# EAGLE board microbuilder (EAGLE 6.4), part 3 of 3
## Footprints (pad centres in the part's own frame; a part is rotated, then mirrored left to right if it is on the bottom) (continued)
TSSOP28 = smd 0.305 x 0.991: 1 -4.225,-2.918; 2 -3.575,-2.918; 3 -2.925,-2.918; 4 -2.275,-2.918; 5 -1.625,-2.918; 6 -0.975,-2.918; 7 -0.325,-2.918; 8 0.325,-2.918; 9 0.975,-2.918; 10 1.625,-2.918; 11 2.275,-2.918; 12 2.925,-2.918; 13 3.575,-2.918; 14 4.225,-2.918; 15 4.225,2.918; 16 3.575,2.918; 17 2.925,2.918; 18 2.275,2.918; 19 1.625,2.918; 20 0.975,2.918; 21 0.325,2.918; 22 -0.325,2.918; 23 -0.975,2.918; 24 -1.625,2.918; 25 -2.275,2.918; 26 -2.925,2.918; 27 -3.575,2.918; 28 -4.225,2.918
U.FL = smd 2.2 x 1.05: 1 0,1.375; 2 0,-1.375 | smd 1.05 x 1: 3 1.525,0
UG-2832HSWEG02_WRAPUNDER = smd 3.2 x 0.35 bottom: 1 -2.03,-4.03; 2 -2.03,-3.41; 3 -2.03,-2.79; 4 -2.03,-2.17; 5 -2.03,-1.55; 6 -2.03,-0.93; 7 -2.03,-0.31; 8 -2.03,0.31; 9 -2.03,0.93; 10 -2.03,1.55; 11 -2.03,2.17; 12 -2.03,2.79; 13 -2.03,3.41; 14 -2.03,4.03
UG-2832HSWEG04 = smd 2.6 x 0.35: 1 15.8,-4.55; 2 15.8,-3.9; 3 15.8,-3.25; 4 15.8,-2.6; 5 15.8,-1.95; 6 15.8,-1.3; 7 15.8,-0.65; 8 15.8,0; 9 15.8,0.65; 10 15.8,1.3; 11 15.8,1.95; 12 15.8,2.6; 13 15.8,3.25; 14 15.8,3.9; 15 15.8,4.55
UG-2832HSWEG04_WRAPAROUND = smd 2.6 x 0.35 bottom: 1 -7.7,-4.55; 2 -7.7,-3.9; 3 -7.7,-3.25; 4 -7.7,-2.6; 5 -7.7,-1.95; 6 -7.7,-1.3; 7 -7.7,-0.65; 8 -7.7,0; 9 -7.7,0.65; 10 -7.7,1.3; 11 -7.7,1.95; 12 -7.7,2.6; 13 -7.7,3.25; 14 -7.7,3.9; 15 -7.7,4.55 | hole 0.8: -2.4,4.625; -2.4,-4.625
UG-2864HSWEG01_0.96IN_WRAPAROUND = smd 0.35 x 2.2 bottom: 1 -10.15,-1.2; 2 -9.45,-1.2; 3 -8.75,-1.2; 4 -8.05,-1.2; 5 -7.35,-1.2; 6 -6.65,-1.2; 7 -5.95,-1.2; 8 -5.25,-1.2; 9 -4.55,-1.2; 10 -3.85,-1.2; 11 -3.15,-1.2; 12 -2.45,-1.2; 13 -1.75,-1.2; 14 -1.05,-1.2; 15 -0.35,-1.2; 16 0.35,-1.2; 17 1.05,-1.2; 18 1.75,-1.2; 19 2.45,-1.2; 20 3.15,-1.2; 21 3.85,-1.2; 22 4.55,-1.2; 23 5.25,-1.2; 24 5.95,-1.2; 25 6.65,-1.2; 26 7.35,-1.2; 27 8.05,-1.2; 28 8.75,-1.2; 29 9.45,-1.2; 30 10.15,-1.2 | hole 0.4: -8,-5.45; 8,-5.45
UG-2864HSWEG01_1.3_WRAPAROUND = smd 0.35 x 2.2 bottom: 1 -10.15,-0.2; 2 -9.45,-0.2; 3 -8.75,-0.2; 4 -8.05,-0.2; 5 -7.35,-0.2; 6 -6.65,-0.2; 7 -5.95,-0.2; 8 -5.25,-0.2; 9 -4.55,-0.2; 10 -3.85,-0.2; 11 -3.15,-0.2; 12 -2.45,-0.2; 13 -1.75,-0.2; 14 -1.05,-0.2; 15 -0.35,-0.2; 16 0.35,-0.2; 17 1.05,-0.2; 18 1.75,-0.2; 19 2.45,-0.2; 20 3.15,-0.2; 21 3.85,-0.2; 22 4.55,-0.2; 23 5.25,-0.2; 24 5.95,-0.2; 25 6.65,-0.2; 26 7.35,-0.2; 27 8.05,-0.2; 28 8.75,-0.2; 29 9.45,-0.2; 30 10.15,-0.2 | hole 0.4: -8,-4.45; 8,-4.45
UG-9616GLBBG02 = smd 3.5 x 0.254: 1 8.25,-3.25; 2 8.25,-2.75; 3 8.25,-2.25; 4 8.25,-1.75; 5 8.25,-1.25; 6 8.25,-0.75; 7 8.25,-0.25; 8 8.25,0.25; 9 8.25,0.75; 10 8.25,1.25; 11 8.25,1.75; 12 8.25,2.25; 13 8.25,2.75; 14 8.25,3.25
UG-9616GLBBG02_0.65MM_WRAPAROUND = smd 3.5 x 0.3 bottom: 1 -5.75,-4.225; 2 -5.75,-3.575; 3 -5.75,-2.925; 4 -5.75,-2.275; 5 -5.75,-1.625; 6 -5.75,-0.975; 7 -5.75,-0.325; 8 -5.75,0.325; 9 -5.75,0.975; 10 -5.75,1.625; 11 -5.75,2.275; 12 -5.75,3.575; 13 -5.75,2.925; 14 -5.75,4.225
UG-9616GLBBG02_WRAPAROUND = smd 3.5 x 0.254 bottom: 1 -3.75,-3.25; 2 -3.75,-2.75; 3 -3.75,-2.25; 4 -3.75,-1.75; 5 -3.75,-1.25; 6 -3.75,-0.75; 7 -3.75,-0.25; 8 -3.75,0.25; 9 -3.75,0.75; 10 -3.75,1.25; 11 -3.75,1.75; 12 -3.75,2.25; 13 -3.75,2.75; 14 -3.75,3.25
UG-9664HDDAG01 = smd 0.4 x 3: 1 -7.7,0.7; 2 -7,0.7; 3 -6.3,0.7; 4 -5.6,0.7; 5 -4.9,0.7; 6 -4.2,0.7; 7 -3.5,0.7; 8 -2.8,0.7; 9 -2.1,0.7; 10 -1.4,0.7; 11 -0.7,0.7; 12 0,0.7; 13 0.7,0.7; 14 1.4,0.7; 15 2.1,0.7; 16 2.8,0.7; 17 3.5,0.7; 18 4.2,0.7; 19 4.9,0.7; 20 5.6,0.7; 21 6.3,0.7; 22 7,0.7; 23 7.7,0.7
UG-9664HDDAG01_WRAPAROUND = smd 0.35 x 3 bottom: 1 -7.7,4.9; 2 -7,4.9; 3 -6.3,4.9; 4 -5.6,4.9; 5 -4.9,4.9; 6 -4.2,4.9; 7 -3.5,4.9; 8 -2.8,4.9; 9 -2.1,4.9; 10 -1.4,4.9; 11 -0.7,4.9; 12 0,4.9; 13 0.7,4.9; 14 1.4,4.9; 15 2.1,4.9; 16 2.8,4.9; 17 3.5,4.9; 18 4.2,4.9; 19 4.9,4.9; 20 5.6,4.9; 21 6.3,4.9; 22 7,4.9; 23 7.7,4.9 | hole 1: -8,1.45; 8,1.45
UG-9664HDDAG01_WRAPAROUND_NOHOLES = smd 0.35 x 3 bottom: 1 -7.7,4.9; 2 -7,4.9; 3 -6.3,4.9; 4 -5.6,4.9; 5 -4.9,4.9; 6 -4.2,4.9; 7 -3.5,4.9; 8 -2.8,4.9; 9 -2.1,4.9; 10 -1.4,4.9; 11 -0.7,4.9; 12 0,4.9; 13 0.7,4.9; 14 1.4,4.9; 15 2.1,4.9; 16 2.8,4.9; 17 3.5,4.9; 18 4.2,4.9; 19 4.9,4.9; 20 5.6,4.9; 21 6.3,4.9; 22 7,4.9; 23 7.7,4.9
UMAX10 = smd 0.29 x 0.9: 1 -1,-2.25; 2 -0.5,-2.25; 3 0,-2.25; 4 0.5,-2.25; 5 1,-2.25; 6 1,2.25; 7 0.5,2.25; 8 0,2.25; 9 -0.5,2.25; 10 -1,2.25
USB-MINIB = smd 0.5 x 2.308: D+ 0,4.064; D- -0.8,4.064; GND 1.6,4.064; ID 0.8,4.064; VBUS -1.6,4.064 | smd 2 x 2.4: GND1 -4.4,-2; GND2 -4.4,3.5; GND3 4.4,3.5; GND4 4.4,-2 | hole 1: -2.2,1; 2.2,1
USB-MINIB_LARGER = smd 0.5 x 2.308: D+ 0,4.064; D- -0.8,4.064; GND 1.6,4.064; ID 0.8,4.064; VBUS -1.6,4.064 | smd 2.54 x 3.81: GND1 -4.4,-2; GND4 4.4,-2 | smd 2 x 2.4: GND2 -4.4,3.5; GND3 4.4,3.5 | hole 1: -2.2,1; 2.2,1
USB_A-SMT = drill 2.5 pad 3.302: D1 -5.85,2.958; D2 5.85,2.958 | drill 1: D3 -2.25,3; D4 2.25,3 | smd 0.8 x 2.5: D+ 1,0; D- -1,0; GND 3.5,0; VBUS -3.5,0
USB_HOST-PTH = drill 0.95 long: D+ 1,6.52; D- -1,6.52; GND 3.5,6.52; VBUS -3.5,6.52 | drill 2.3 pad 2.9: S1 -6.57,3.81; S2 6.57,3.81
VCNL4000 = smd 0.35 x 0.805: 1 -1.5,-1.772; 2 -0.75,-1.772; 3 0,-1.772; 4 0.75,-1.772; 5 1.5,-1.772; 7 1.5,1.772; 8 0.75,1.772; 9 0,1.772; 10 -0.75,1.772; 11 -1.5,1.772 | smd 0.805 x 0.4: 6 1.772,-0.715; 12 -1.772,-0.2
VFBGA54 = smd 0.34 x 0.34: A1 -3.2,3.2; A2 -2.4,3.2; A3 -1.6,3.2; A7 1.6,3.2; A8 2.4,3.2; A9 3.2,3.2; B1 -3.2,2.4; B2 -2.4,2.4; B3 -1.6,2.4; B7 1.6,2.4; B8 2.4,2.4; B9 3.2,2.4; C1 -3.2,1.6; C2 -2.4,1.6; C3 -1.6,1.6; C7 1.6,1.6; C8 2.4,1.6; C9 3.2,1.6; D1 -3.2,0.8; D2 -2.4,0.8; D3 -1.6,0.8; D7 1.6,0.8; D8 2.4,0.8; D9 3.2,0.8; E1 -3.2,0; E2 -2.4,0; E3 -1.6,0; E7 1.6,0; E8 2.4,0; E9 3.2,0; F1 -3.2,-0.8; F2 -2.4,-0.8; F3 -1.6,-0.8; F7 1.6,-0.8; F8 2.4,-0.8; F9 3.2,-0.8; G1 -3.2,-1.6; G2 -2.4,-1.6; G3 -1.6,-1.6; G7 1.6,-1.6; G8 2.4,-1.6; G9 3.2,-1.6; H1 -3.2,-2.4; H2 -2.4,-2.4; H3 -1.6,-2.4; H7 1.6,-2.4; H8 2.4,-2.4; H9 3.2,-2.4; J1 -3.2,-3.2; J2 -2.4,-3.2; J3 -1.6,-3.2; J7 1.6,-3.2; J8 2.4,-3.2; J9 3.2,-3.2
VFSOP-8 = smd 0.25 x 0.65: 1 -0.75,-1.45; 2 -0.25,-1.45; 3 0.25,-1.45; 4 0.75,-1.45; 5 0.75,1.45; 6 0.25,1.45; 7 -0.25,1.45; 8 -0.75,1.45
WFDFN-14 = smd 0.2 x 0.6: P$1 -1.2,-1.5; P$2 -0.8,-1.5; P$3 -0.4,-1.5; P$4 0,-1.5; P$5 0.4,-1.5; P$6 0.8,-1.5; P$7 1.2,-1.5; P$8 1.2,1.5; P$9 0.8,1.5; P$10 0.4,1.5; P$11 0,1.5; P$12 -0.4,1.5; P$13 -0.8,1.5; P$14 -1.2,1.5 | smd 2.3 x 1.7: P$THERM 0,0
WLCSP16 = smd 0.35 x 0.35: A1 -0.75,0.75; A2 -0.25,0.75; A3 0.25,0.75; A4 0.75,0.75; B1 -0.75,0.25; B2 -0.25,0.25; B3 0.25,0.25; B4 0.75,0.25; C1 -0.75,-0.25; C2 -0.25,-0.25; C3 0.25,-0.25; C4 0.75,-0.25; D1 -0.75,-0.75; D2 -0.25,-0.75; D3 0.25,-0.75; D4 0.75,-0.75
WQFN16 = smd 0.28 x 0.85: P$1 -0.75,-1.475; P$2 -0.25,-1.475; P$3 0.25,-1.475; P$4 0.75,-1.475; P$9 0.75,1.475; P$10 0.25,1.475; P$11 -0.25,1.475; P$12 -0.75,1.475 | smd 0.85 x 0.28: P$5 1.475,-0.75; P$6 1.475,-0.25; P$7 1.475,0.25; P$8 1.475,0.75; P$13 -1.475,0.75; P$14 -1.475,0.25; P$15 -1.475,-0.25; P$16 -1.475,-0.75 | smd 1.65 x 1.65: P$17 0,0
WQFN20 = smd 0.28 x 0.85: 1 -1,-1.975; 2 -0.5,-1.975; 3 0,-1.975; 4 0.5,-1.975; 5 1,-1.975; 11 1,1.975; 12 0.5,1.975; 13 0,1.975; 14 -0.5,1.975; 15 -1,1.975 | smd 0.85 x 0.28: 6 1.975,-1; 7 1.975,-0.5; 8 1.975,0; 9 1.975,0.5; 10 1.975,1; 16 -1.975,1; 17 -1.975,0.5; 18 -1.975,0; 19 -1.975,-0.5; 20 -1.975,-1 | smd 2.65 x 2.65: 21 0,0
XBEE = drill 0.8 pad 1.27: 1 -11,9; 2 -11,7; 3 -11,5; 4 -11,3; 5 -11,1; 6 -11,-1; 7 -11,-3; 8 -11,-5; 9 -11,-7; 10 -11,-9; 11 11,-9; 12 11,-7; 13 11,-5; 14 11,-3; 15 11,-1; 16 11,1; 17 11,3; 18 11,5; 19 11,7; 20 11,9
XBEE-PRO = drill 0.8 pad 1.27: 1 -11,9; 2 -11,7; 3 -11,5; 4 -11,3; 5 -11,1; 6 -11,-1; 7 -11,-3; 8 -11,-5; 9 -11,-7; 10 -11,-9; 11 11,-9; 12 11,-7; 13 11,-5; 14 11,-3; 15 11,-1; 16 11,1; 17 11,3; 18 11,5; 19 11,7; 20 11,9
_0402 = smd 0.6 x 0.6: 1 -0.508,0; 2 0.508,0
_0402MP = smd 0.5 x 0.5: 1 -0.508,0; 2 0.508,0
_0603 = smd 0.9 x 0.8: 1 -0.762,0; 2 0.762,0
_0603MP = smd 0.8 x 0.8: 1 -0.762,0; 2 0.762,0
_0805 = smd 1.2 x 1.3: 1 -1.016,0; 2 1.016,0
_0805MP = smd 1.2 x 1.3: 1 -1.016,0; 2 1.016,0

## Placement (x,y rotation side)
0  [1X01_2MM]  not placed on the board
1  [1X01_2MM_OVAL]  not placed on the board
2  [1X01_OVAL]  not placed on the board
3  [1X01_ROUND]  not placed on the board
4  [1X02_OVAL]  not placed on the board
5  [1X02_ROUND]  not placed on the board
6  [1X02_SMT]  not placed on the board
7  [1X03_1.0MM]  not placed on the board
8  [1X03_OVAL]  not placed on the board
9  [1X03_ROUND]  not placed on the board
10  [1X03_ROUND_76]  not placed on the board
11  [1X03_SMT]  not placed on the board
12  [1X04_1.0MM]  not placed on the board
13  [1X04_OVAL]  not placed on the board
14  [1X04_ROUND]  not placed on the board
15  [1X04_ROUND_76]  not placed on the board
16  [1X04_SMT]  not placed on the board
17  [1X05_1.27MM]  not placed on the board
18  [1X05_OVAL]  not placed on the board
19  [1X05_ROUND]  not placed on the board
20  [1X05_ROUND_70]  not placed on the board
21  [1X05_ROUND_76]  not placed on the board
22  [1X05_SMT]  not placed on the board
23  [1X06_OVAL]  not placed on the board
24  [1X06_ROUND]  not placed on the board
25  [1X06_ROUND_70]  not placed on the board
26  [1X06_ROUND_76]  not placed on the board
27  [1X06_SMT]  not placed on the board
28  [1X07_OVAL]  not placed on the board
29  [1X07_ROUND]  not placed on the board
30  [1X07_ROUND_70]  not placed on the board
31  [1X07_ROUND_76]  not placed on the board
32  [1X08_OVAL]  not placed on the board
33  [1X08_ROUND]  not placed on the board
34  [1X08_ROUND_70]  not placed on the board
35  [1X08_ROUND_76]  not placed on the board
36  [1X09_OVAL]  not placed on the board
37  [1X09_ROUND_70]  not placed on the board
38  [1X09_ROUND_76]  not placed on the board
39  [1X10_OVAL]  not placed on the board
40  [1X10_ROUND]  not placed on the board
41  [1X10_ROUND70]  not placed on the board
42  [1X10_ROUND_2MM]  not placed on the board
43  [1X10_ROUND_76]  not placed on the board
44  [1X10_SMT]  not placed on the board
45  [1X11_ROUND]  not placed on the board
46  [1X11_ROUND_76]  not placed on the board
47  [1X12_OVAL]  not placed on the board
48  [1X12_ROUND]  not placed on the board
49  [1X12_ROUND_76MIL]  not placed on the board
50  [1X12_ROUND_80MIL]  not placed on the board
51  [1X13_ROUND_70]  not placed on the board
52  [1X15_ROUND_70]  not placed on the board
53  [1X16_2MM]  not placed on the board
54  [1X16_2MM_OVAL]  not placed on the board
55  [1X16_OVAL]  not placed on the board
56  [1X16_ROUND]  not placed on the board
57  [1X17_ROUND70]  not placed on the board
58  [1X20_ROUND]  not placed on the board
59  [1X23_ROUND_70MIL]  not placed on the board
60  [1X27_OVAL]  not placed on the board
61  [1X27_ROUND]  not placed on the board
62  [1X28_OVAL]  not placed on the board
63  [2X03_ROUND_70MIL]  not placed on the board
64  [2X05]  not placed on the board
65  [2X05_1.27MM_SMT]  not placed on the board
66  [2X07]  not placed on the board
67  [2X08]  not placed on the board
68  [2X10]  not placed on the board
69  [2X13]  not placed on the board
70  [2X15]  not placed on the board
71  [2X16]  not placed on the board
72  [2X23]  not placed on the board
73  [3X04]  not placed on the board
74  [3X08]  not placed on the board
75  [4UCONN_05550]  not placed on the board
76  [4UCONN_19269]  not placed on the board
77  [4UCONN_19621]  not placed on the board
78  [4UCONN_19621_SPARK]  not placed on the board
79  [32QN2]  not placed on the board
80  [869MHZANTENNA]  not placed on the board
81  [0402]  not placed on the board
82  [0603]  not placed on the board
83  [0603-MINI]  not placed on the board
84  [0805]  not placed on the board
85  [0805-THM]  not placed on the board
86  [0805_NOTHERMALS]  not placed on the board
87  [1206]  not placed on the board
88  [2012]  not placed on the board
89  [2512]  not placed on the board
90  [ADAFRUIT_2.5MM]  not placed on the board
91  [ADAFRUIT_3.5MM]  not placed on the board
92  [ADAFRUIT_5MM]  not placed on the board
93  [ADAFRUIT_9MM]  not placed on the board
94  [ADAFRUIT_16MM]  not placed on the board
95  [ADAFRUIT_30MM]  not placed on the board
96  [ADAFRUIT_TEXT_20MM]  not placed on the board
97  [ADAFRUIT_TEXT_30MM]  not placed on the board
98  [ADBM-A350]  not placed on the board
99  [ALTOIDSMINTS]  not placed on the board
100  [ANT_868MHZ_SPLATCH]  0,0 0 top
101  [ARDUINO]  25.4,0 0 top
102  [ARDUINO-NODIM]  50.8,0 0 top
103  [ARDUINO-NOHOLE]  76.2,0 0 top
104  [ARDUINOR3]  101.6,0 0 top
105  [ARDUINOR3-BPLACE]  127,0 0 top
106  [ARDUINOR3-NODIM]  152.4,0 0 top
107  [BALUN0603]  177.8,0 0 top
108  [BALUN0805]  203.2,0 0 top
109  [BALUN1206]  228.6,0 0 top
110  [BATTOUTLINE_LIPO1300MAH]  0,25.4 0 top
111  [BATTOUTLINE_LIPO2700MAH]  25.4,25.4 0 top
112  [BEAGLEBONE_SHIELD]  50.8,25.4 0 top
113  [BLUETOOTH_MODULE]  76.2,25.4 0 top
114  [BMC050]  101.6,25.4 0 top
115  [BMC050_EXTENDED]  127,25.4 0 top
116  [BMI-S-202-F]  152.4,25.4 0 top
117  [BMI-S-209-F]  177.8,25.4 0 top
118  [BMP085]  203.2,25.4 0 top
119  [BREAKOUT_SOIC8]  228.6,25.4 0 top
120  [BREAKOUT_SOIC24]  0,50.8 0 top
121  [BREAKOUT_SOT23-6]  25.4,50.8 0 top
122  [BTL221722-276L]  50.8,50.8 0 top
123  [BTN_EVQPQ_4.5MM]  76.2,50.8 0 top
124  [BTN_KMR2_4.6X2.8]  101.6,50.8 0 top
125  [BUS_ADC_5MM]  127,50.8 0 top
126  [BUS_I2C_5MM]  152.4,50.8 0 top
127  [BUS_SPI_5MM]  177.8,50.8 0 top
128  [C707_10M006_512_2]  203.2,50.8 0 top
129  [CELEC_3.5MM_8MM]  228.6,50.8 0 top
130  [CELEC_3.5MM_10MM]  0,76.2 0 top
131  [CFAF240320K-T-TS]  25.4,76.2 0 top
132  [CHIPLED_0603]  50.8,76.2 0 top
133  [CHIPLED_0603_NOOUTLINE]  76.2,76.2 0 top
134  [CHIPLED_0805]  101.6,76.2 0 top
135  [CHIPLED_0805_NOOUTLINE]  127,76.2 0 top
136  [CHIPLED_1206]  152.4,76.2 0 top
137  [CORTEXM3_SWD10_MOLEX]  177.8,76.2 0 top
138  [CR1220]  203.2,76.2 0 top
139  [CR2032]  228.6,76.2 0 top
140  [CRYSTAL_2.5X2]  0,101.6 0 top
141  [CRYSTAL_3.2X2.5]  25.4,101.6 0 top
142  [CRYSTAL_4.9X1.8]  50.8,101.6 0 top
143  [CRYSTAL_8X3.8]  76.2,101.6 0 top
144  [CRYSTAL_CYL_2X6MM_SMT]  101.6,101.6 0 top
145  [DCJACK_1.3MM_PTH]  127,101.6 0 top
146  [DCJACK_2MM_PTH]  152.4,101.6 0 top
147  [DCJACK_2MM_SMT]  177.8,101.6 0 top
148  [DFN10_3X3MM]  203.2,101.6 0 top
149  [DFN14_4X3MM]  228.6,101.6 0 top
150  [DIL08]  0,127 0 top
151  [DIL28_600MIL]  25.4,127 0 top
152  [DIL40_0.9]  50.8,127 0 top
153  [DIPSWITCH_2PIN]  76.2,127 0 top
154  [DIRECTION_BIDIR]  101.6,127 0 top
155  [DIRECTION_IN]  127,127 0 top
156  [DIRECTION_OUT]  152.4,127 0 top
157  [DO-1N4148]  177.8,127 0 top
158  [DPDT_SMT_JS202011SCQN]  203.2,127 0 top
159  [EIA3216-18/A-R]  228.6,127 0 top
160  [EIA3216-18/A-W]  0,152.4 0 top
161  [EIA3528-21/B-R]  25.4,152.4 0 top
162  [EIA3528-21/B-W]  50.8,152.4 0 top
163  [EIA6032-28/C-R]  76.2,152.4 0 top
164  [EIA6032-28/C-W]  101.6,152.4 0 top
165  [EIA7343-31/D-R]  127,152.4 0 top
166  [EIA7343-31/D-W]  152.4,152.4 0 top
167  [EINK_10BAR]  177.8,152.4 0 top
168  [ENCLOSURE_SS125]  203.2,152.4 0 top
169  [ENCLOSURE_TB55]  228.6,152.4 0 top
170  [ENCLOSURE_TB56]  0,177.8 0 top
171  [ENCLOSURE_TB59]  25.4,177.8 0 top
172  [ENCLOSURE_WINDOW_82X60X20]  50.8,177.8 0 top
173  [EVQ-Q2]  76.2,177.8 0 top
174  [FGPMMOPA6B]  101.6,177.8 0 top
175  [FGPMMOPA6C]  127,177.8 0 top
176  [FGPMMOPA6H]  152.4,177.8 0 top
177  [FH26-17S-0.3SHW]  177.8,177.8 0 top
178  [FIDUCIAL-1.5X3]  203.2,177.8 0 top
179  [FIDUCIAL-1X2]  228.6,177.8 0 top
180  [FIDUCIAL-1X2.5]  0,203.2 0 top
181  [FIDUCIAL_1MM]  25.4,203.2 0 top
182  [FPC4PIN]  50.8,203.2 0 top
183  [FPC40PIN]  76.2,203.2 0 top
184  [FPC45PIN]  101.6,203.2 0 top
185  [FPC_10PIN_52892-1095]  127,203.2 0 top
186  [FPC_XF2M-3015-1A]  152.4,203.2 0 top
187  [GE864]  177.8,203.2 0 top
188  [GE865]  203.2,203.2 0 top
189  [GM862]  228.6,203.2 0 top
190  [GM862_CONNECTOR]  0,228.6 0 top
191  [HB100]  25.4,228.6 0 top
192  [HC49UP]  50.8,228.6 0 top
193  [HDMI_MOLEX_47151-0001]  76.2,228.6 0 top
194  [HEADER_1X02]  101.6,228.6 0 top
195  [HEADER_1X05]  127,228.6 0 top
196  [HMC5883L]  152.4,228.6 0 top
197  [HMC5883L_EXTENDED]  177.8,228.6 0 top
198  [HTSSOP16]  203.2,228.6 0 top
199  [HVQFN32]  228.6,228.6 0 top
200  [HVQFN32-5X5]  0,254 0 top
201  [HVQFN32-5X5_3MMTHERMAL]  25.4,254 0 top
202  [HVQFN33-7X7]  50.8,254 0 top
203  [HVQFN40-6X6]  76.2,254 0 top
204  [HVQFN64]  101.6,254 0 top
205  [ILI9325_28INCH_TS]  127,254 0 top
206  [ILI9325_28INCH_TS_OUTLINE]  152.4,254 0 top
207  [ILI9481_35INCH_OUTLINE]  177.8,254 0 top
208  [INDUCTOR_5X5MM_NR5040_NOTHERMALS]  203.2,254 0 top
209  [INDUCTOR_5X5MM_TDK_VLC5045]  228.6,254 0 top
210  [INDUCTOR_5X5MM_TDK_VLC5045_NOTHERMALS]  0,279.4 0 top
211  [INDUCTOR_6X6MM_TDK_SLF6045]  25.4,279.4 0 top
212  [INDUCTOR_6X6MM_TDK_VLC6045]  50.8,279.4 0 top
213  [INDUCTOR_1007]  76.2,279.4 0 top
214  [ITG3200_QFN24]  101.6,279.4 0 top
215  [JD-T1800]  127,279.4 0 top
216  [JSTPH2]  152.4,279.4 0 top
217  [JSTPH2_NOTHERMALS]  177.8,279.4 0 top
218  [JSTPH3]  203.2,279.4 0 top
219  [JSTPH4]  228.6,279.4 0 top
220  [JSTPH6]  0,304.8 0 top
221  [JSTPH8]  25.4,304.8 0 top
222  [JSTSH2]  50.8,304.8 0 top
223  [JTAG-ARM]  76.2,304.8 0 top
224  [JUMPER2]  101.6,304.8 0 top
225  [JUMPER3]  127,304.8 0 top
226  [L3G4200D_LGA16L]  152.4,304.8 0 top
227  [LBGA256_1.0MM]  177.8,304.8 0 top
228  [LFCSP16-R]  203.2,304.8 0 top
229  [LFCSP16-W]  228.6,304.8 0 top
230  [LGA8]  0,330.2 0 top
231  [LGA14]  25.4,330.2 0 top
232  [LGA16_3X3MM]  50.8,330.2 0 top
233  [LGA16_5X5MM]  76.2,330.2 0 top
234  [LLP40]  101.6,330.2 0 top
235  [LOGIC_3.3V_5MM]  127,330.2 0 top
236  [LOGIC_5VREADY_5MM]  152.4,330.2 0 top
237  [LOGIC_5V_5MM]  177.8,330.2 0 top
238  [LOWPASSFILTER0603]  203.2,330.2 0 top
239  [LQFP48]  228.6,330.2 0 top
240  [LQFP64]  0,355.6 0 top
241  [LQFP80]  25.4,355.6 0 top
242  [LQFP100]  50.8,355.6 0 top
243  [LQFP144]  76.2,355.6 0 top
244  [LQFP208]  101.6,355.6 0 top
245  [MICROSD]  127,355.6 0 top
246  [MINIMOLD6]  152.4,355.6 0 top
247  [MOLEX20_RIGHTANGLE]  177.8,355.6 0 top
248  [MOUNTINGHOLE_1.0_PLATED]  203.2,355.6 0 top
249  [MOUNTINGHOLE_2.0_PLATED]  228.6,355.6 0 top
250  [MOUNTINGHOLE_2.5_PLATED]  0,381 0 top
251  [MOUNTINGHOLE_2.5_PLATED_THICK]  25.4,381 0 top
252  [MOUNTINGHOLE_2.8]  50.8,381 0 top
253  [MOUNTINGHOLE_3.0]  76.2,381 0 top
254  [MOUNTINGHOLE_3.0_PLATED]  101.6,381 0 top
255  [MOUNTINGHOLE_3.0_PLATEDTHIN]  127,381 0 top
256  [MOUNTINGHOLE_3.2]  152.4,381 0 top
257  [MSOP8_0.65MM]  177.8,381 0 top
258  [MSOP10]  203.2,381 0 top
259  [OSC_3.2X2.5MM]  228.6,381 0 top
260  [OSC_7X5MM]  0,406.4 0 top
261  [PAD-1.5X2.0]  25.4,406.4 0 top
262  [PANASONIC_C]  50.8,406.4 0 top
263  [PANASONIC_D]  76.2,406.4 0 top
264  [PASS-ROUND]  101.6,406.4 0 top
265  [POWER_3.3-5.0V_5MM]  127,406.4 0 top
266  [PSP_BACKLIGHTCON]  152.4,406.4 0 top
267  [PSP_LCDOUTLINE]  177.8,406.4 0 top
268  [PSP_TSCON]  203.2,406.4 0 top
269  [PTC1210]  228.6,406.4 0 top
270  [PTC1812]  0,431.8 0 top
271  [PUSHBUTTON_SMD_SJ]  25.4,431.8 0 top
272  [QFN16_3MM]  50.8,431.8 0 top
273  [QFN20_3MM]  76.2,431.8 0 top
274  [QFN20_4MM]  101.6,431.8 0 top
275  [QFN24_4MM]  127,431.8 0 top
276  [QFN28_5MM]  152.4,431.8 0 top
277  [QFN32_5MM]  177.8,431.8 0 top
278  [QSOP24_0.635MM]  203.2,431.8 0 top
279  [RASBERRYPI_IDC]  228.6,431.8 0 top
280  [RASBERRYPI_SHIELD]  0,457.2 0 top
281  [RESPACK_4X0603]  25.4,457.2 0 top
282  [RGBLED_PLCC4]  50.8,457.2 0 top
283  [RGBLED_PLCC6]  76.2,457.2 0 top
284  [RJ45PTH]  101.6,457.2 0 top
285  [RJ45SMT]  127,457.2 0 top
286  [RJ45_PULSEJACK]  152.4,457.2 0 top
287  [S6B33B6_1.5IN_LCD]  177.8,457.2 0 top
288  [SC70-6L]  203.2,457.2 0 top
289  [SDCARD_PCBCARRIER_DIM]  228.6,457.2 0 top
290  [SDCARD_PCBCARRIER_DOCU]  0,482.6 0 top
291  [SDCARD_SMT_4U06132]  25.4,482.6 0 top
292  [SDCARD_SMT_4U19646]  50.8,482.6 0 top
293  [SEGMENT-BL-Q56C43]  76.2,482.6 0 top
294  [SEGMENT_BICOL_BL-AR12Z3010]  101.6,482.6 0 top
295  [SEGMENT_BICOL_BL-M12A883XX]  127,482.6 0 top
296  [SEGMENT_BL-M07C881UR]  152.4,482.6 0 top
297  [SEGMENT_BL-M12A881UR]  177.8,482.6 0 top
298  [SEGMENT_BL-M12A883]  203.2,482.6 0 top
299  [SEGMENT_BL-Q39A-42]  228.6,482.6 0 top
300  [SEGMENT_STARBURST_BL-S80A-13]  0,508 0 top
301  [SEGMENT_STARBURST_BL-S230B-12]  25.4,508 0 top
302  [SI473X_SSOP]  50.8,508 0 top
303  [SIM900B_SMT]  76.2,508 0 top
304  [SIM900_SMT]  101.6,508 0 top
305  [SIM908]  127,508 0 top
306  [SIM_5002]  152.4,508 0 top
307  [SMA90_DIP]  177.8,508 0 top
308  [SMADIODE]  203.2,508 0 top
309  [SMB_DIP]  228.6,508 0 top
310  [SOCKET_LBGA256_8117-256-4E-01]  0,533.4 0 top
311  [SOD-123]  25.4,533.4 0 top
312  [SOD-323]  50.8,533.4 0 top
313  [SOD-523]  76.2,533.4 0 top
314  [SOIC-4]  101.6,533.4 0 top
315  [SOIC8_150MIL]  127,533.4 0 top
316  [SOIC8_208MIL]  152.4,533.4 0 top
317  [SOIC14]  177.8,533.4 0 top
318  [SOIC16]  203.2,533.4 0 top
319  [SOIC20WIDE]  228.6,533.4 0 top
320  [SOIC24WIDE]  0,558.8 0 top
321  [SOLDERJUMPER_2WAY_OPEN_0603]  25.4,558.8 0 top
322  [SOLDERJUMPER_2WAY_OPEN_0805]  50.8,558.8 0 top
323  [SOLDERJUMPER_2WAY_OPEN_NOPASTE]  76.2,558.8 0 top
324  [SOLDERJUMPER_ARROW_NOPASTE]  101.6,558.8 0 top
325  [SOLDERJUMPER_CLOSEDPERM]  127,558.8 0 top
326  [SOLDERJUMPER_CLOSEDWIRE]  152.4,558.8 0 top
327  [SOLDERJUMPER_REFLOW]  177.8,558.8 0 top
328  [SOLDERJUMPER_REFLOW_NOPASTE]  203.2,558.8 0 top
329  [SOLDERJUMPER_WAVE]  228.6,558.8 0 top
330  [SOP8-1351]  0,584.2 0 top
331  [SOP8-1369]  25.4,584.2 0 top
332  [SOP20_300MIL]  50.8,584.2 0 top
333  [SOP24_300MIL]  76.2,584.2 0 top
334  [SOP28_300MIL]  101.6,584.2 0 top
335  [SOT23-5]  127,584.2 0 top
336  [SOT23-6]  152.4,584.2 0 top
337  [SOT23-8]  177.8,584.2 0 top
338  [SOT23-R]  203.2,584.2 0 top
339  [SOT23-W]  228.6,584.2 0 top
340  [SOT23-WIDE]  0,609.6 0 top
341  [SOT223-R]  25.4,609.6 0 top
342  [SOT223-W]  50.8,609.6 0 top
343  [SOT323-R]  76.2,609.6 0 top
344  [SOT323-W]  101.6,609.6 0 top
345  [SOT363]  127,609.6 0 top
346  [SOT833-1]  152.4,609.6 0 top
347  [SOT886]  177.8,609.6 0 top
348  [SPDT_SMT_SSSS811101]  203.2,609.6 0 top
349  [SPST_SMT_19192]  228.6,609.6 0 top
350  [SSOP24]  0,635 0 top
351  [SSOP28DB]  25.4,635 0 top
352  [STANDARDCONNECTOR]  50.8,635 0 top
353  [STX3100]  76.2,635 0 top
354  [SWITCH_4WAY_TPA511GLFS]  101.6,635 0 top
355  [SYMBOL_GYROXYZ_10MM]  127,635 0 top
356  [TCS3414_CS6]  152.4,635 0 top
357  [TDFN14_3X3MM]  177.8,635 0 top
358  [TEA5767MODULE]  203.2,635 0 top
359  [TERMBLOCK_1X2-3.5MM]  228.6,635 0 top
360  [TERMBLOCK_1X3-3.5MM]  0,660.4 0 top
361  [TESTPOINT_PAD_2MM]  25.4,660.4 0 top
362  [TESTPOINT_ROUND_0.5MM]  50.8,660.4 0 top
363  [TESTPOINT_ROUND_1MM]  76.2,660.4 0 top
364  [TESTPOINT_ROUND_2MM]  101.6,660.4 0 top
365  [TESTPOINT_SMT]  127,660.4 0 top
366  [TFBGA100_0.8]  152.4,660.4 0 top
367  [TFBGA180_0.8]  177.8,660.4 0 top
368  [TFBGA208_0.8]  203.2,660.4 0 top
369  [TFBGA208_0.65]  228.6,660.4 0 top
370  [TMLF-6]  0,685.8 0 top
371  [TO92]  25.4,685.8 0 top
372  [TO92-LINE]  50.8,685.8 0 top
373  [TO252]  76.2,685.8 0 top
374  [TO263-5]  101.6,685.8 0 top
375  [TO263-5_NOPASTE]  127,685.8 0 top
376  [TPS851]  152.4,685.8 0 top
377  [TPS61029]  177.8,685.8 0 top
378  [TRIMPOT_BOURNS3MM]  203.2,685.8 0 top
379  [TSL13T]  228.6,685.8 0 top
380  [TSL2561_CS6]  0,711.2 0 top
381  [TSL2561_FN]  25.4,711.2 0 top
382  [TSOP54-400]  50.8,711.2 0 top
383  [TSSOP5]  76.2,711.2 0 top
384  [TSSOP8]  101.6,711.2 0 top
385  [TSSOP8-4.4MM]  127,711.2 0 top
386  [TSSOP14]  152.4,711.2 0 top
387  [TSSOP16]  177.8,711.2 0 top
388  [TSSOP20]  203.2,711.2 0 top
389  [TSSOP28]  228.6,711.2 0 top
390  [U.FL]  0,736.6 0 top
391  [UG-2832HSWEG02_WRAPUNDER]  25.4,736.6 0 top
392  [UG-2832HSWEG04]  50.8,736.6 0 top
393  [UG-2832HSWEG04_WRAPAROUND]  76.2,736.6 0 top
394  [UG-2864HSWEG01_0.96IN_WRAPAROUND]  101.6,736.6 0 top
395  [UG-2864HSWEG01_1.3_WRAPAROUND]  127,736.6 0 top
396  [UG-9616GLBBG02]  152.4,736.6 0 top
397  [UG-9616GLBBG02_0.65MM_WRAPAROUND]  177.8,736.6 0 top
398  [UG-9616GLBBG02_WRAPAROUND]  203.2,736.6 0 top
399  [UG-9664HDDAG01]  228.6,736.6 0 top
400  [UG-9664HDDAG01_WRAPAROUND]  not placed on the board
401  [UG-9664HDDAG01_WRAPAROUND_NOHOLES]  not placed on the board
402  [UMAX10]  not placed on the board
403  [USB-MINIB]  not placed on the board
404  [USB-MINIB_LARGER]  not placed on the board
405  [USB_A-SMT]  not placed on the board
406  [USB_HOST-PTH]  not placed on the board
407  [VCNL4000]  not placed on the board
408  [VFBGA54]  not placed on the board
409  [VFSOP-8]  not placed on the board
410  [WFDFN-14]  not placed on the board
411  [WLCSP16]  not placed on the board
412  [WQFN16]  not placed on the board
413  [WQFN20]  not placed on the board
414  [XBEE]  not placed on the board
415  [XBEE-PRO]  not placed on the board
416  [_0402]  not placed on the board
417  [_0402MP]  not placed on the board
418  [_0603]  not placed on the board
419  [_0603MP]  not placed on the board
420  [_0805]  not placed on the board
421  [_0805MP]  not placed on the board

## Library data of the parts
0 1-421 = microbuilder

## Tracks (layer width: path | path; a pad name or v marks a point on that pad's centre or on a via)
(copper drawn outside any net)
  shapes: Top area x1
